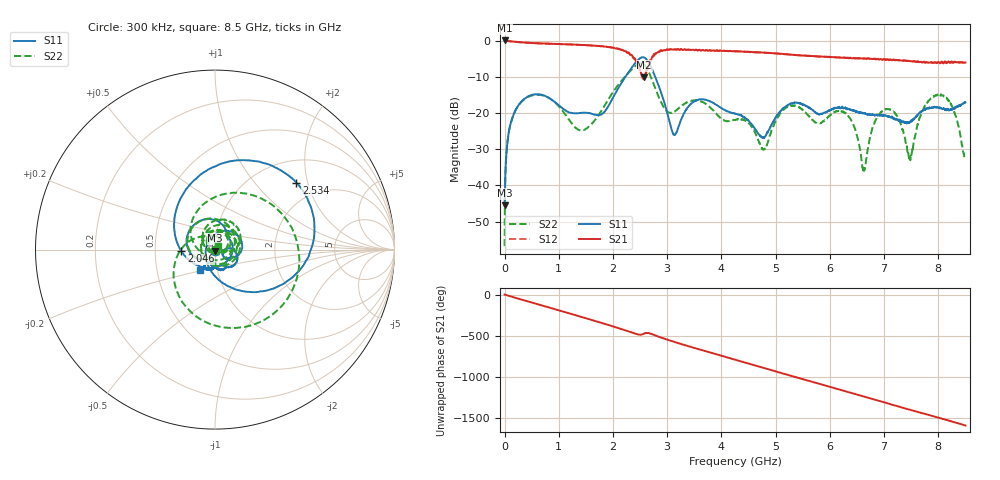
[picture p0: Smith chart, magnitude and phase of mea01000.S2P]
!Agilent Technologies,E5071B,MY42402595,A.08.01
!Date: Tue Jan 02 09:55:01 2001
!Data & Calibration Information:
!Freq	S11:SOLT2(ON)	S21:SOLT2(ON)	S12:SOLT2(ON)	S22:SOLT2(ON)
# Hz S dB R 50
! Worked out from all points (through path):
!   1601 points, 300 kHz to 8.5 GHz, reference 50 ohm
!   highest |S21| = 0.02 dB at 300 kHz (marker M1); lowest = -10.2 dB at 2.577 GHz (marker M2)
!   group delay of S21, straight-line fit = 516 ps
!   lowest |S11| = -45.5 dB at 300 kHz (marker M3), VSWR 1.01, Z = 50.1 - j0.514 ohm
!   |S11| at or under -10 dB: start of sweep to 2.229 GHz; 2.778 GHz to end of sweep
!   |S22| runs from -56.8 to -6.2 dB; largest |S21 - S12| = 0.04
!   S11 on the Smith chart (normalised r, x): 300 kHz: 1.00, -0.01; 2.046 GHz: 0.68, -0.01; 2.534 GHz: 1.50, +1.70; 8.5 GHz: 0.82, -0.19
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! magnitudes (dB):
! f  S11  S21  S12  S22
! 300 kHz  -45.5  0.0  0.0  -56.8
! 79.98 MHz  -25.0  -0.2  -0.2  -25.1
! 319 MHz  -16.7  -0.5  -0.5  -16.8
! 1.419 GHz  -20.0  -1.2  -1.2  -24.8
! 2.046 GHz  -14.5  -2.2  -2.1  -13.2
! 2.534 GHz  -4.6  -9.9  -9.8  -6.3
! 2.577 GHz  -4.7  -10.2  -9.7  -6.6
! 2.837 GHz  -12.3  -3.1  -3.2  -15.4
! 3.129 GHz  -26.0  -2.4  -2.5  -19.6
! 3.554 GHz  -16.5  -2.7  -2.7  -16.5
! 4.25 GHz  -20.1  -3.0  -3.0  -21.9
! 4.776 GHz  -26.8  -3.3  -3.3  -30.1
! 5.19 GHz  -18.1  -3.8  -3.8  -18.5
! 5.669 GHz  -19.1  -4.3  -4.3  -21.7
! 6.306 GHz  -18.8  -4.8  -4.8  -20.3
! 6.625 GHz  -20.0  -5.0  -5.0  -35.6
! 6.832 GHz  -20.7  -5.1  -5.0  -22.4
! 7.087 GHz  -21.0  -5.4  -5.3  -19.0
! 7.475 GHz  -22.5  -5.7  -5.7  -32.4
! 7.762 GHz  -19.1  -6.1  -6.0  -17.8
! 8.107 GHz  -18.7  -6.1  -6.0  -15.3
! 8.5 GHz  -17.1  -6.1  -6.1  -31.9
